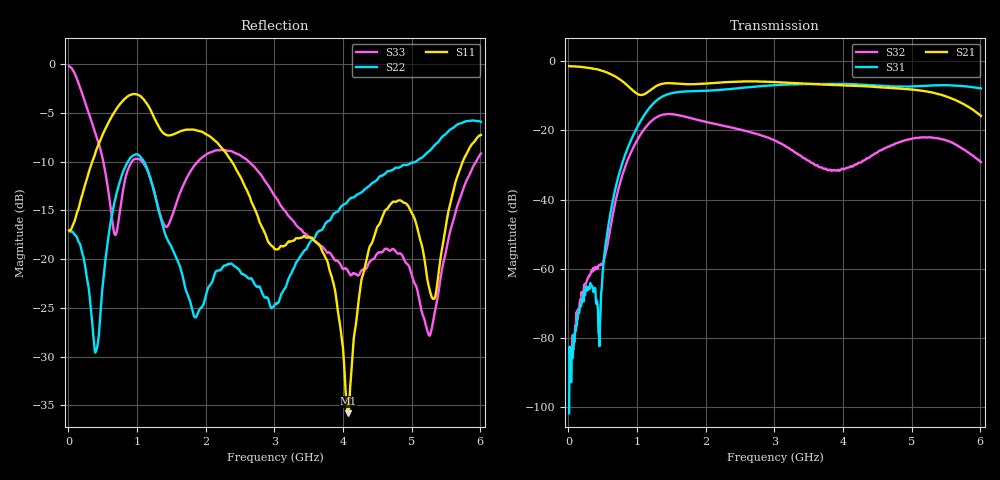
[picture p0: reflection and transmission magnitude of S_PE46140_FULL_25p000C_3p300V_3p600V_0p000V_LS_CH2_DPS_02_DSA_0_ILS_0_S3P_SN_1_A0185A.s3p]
! Device ID: PE46140_FULL
! File Path: z:\PE46140\MajorStates\25p000C\3p300\LS_CH2_DPS_02_DSA_0_ILS_0\PE46140_FULL_25p000C_3p300V_3p600V_0p000V_LS_CH2_DPS_02_DSA_0_ILS_0_S3P_SN_1_A0185A.s3p
! Serial: 1
! Lot: A0185A
! Temp: 25.000C
! VDD: 3.300
! VSS: 0.000
! Control_Hi: 3.600
! Control_Lo: 0.000
! Logic State: LS_CH2_DPS_02_DSA_0_ILS_0
! Port 1: RFIN
! Port 2: RFOUT1
! Port 3: RFOUT2
! ThroughPath:1-3
! IDD: 0.0003146759
! ISS: -1.196e-007
! Comment:
#  Hz  S  RI  R  50
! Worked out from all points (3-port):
!   801 points, 10 MHz to 6.01 GHz, reference 50 ohm
!   strongest paths, dB at 10 MHz, 1.51 GHz, 3.01 GHz, 4.51 GHz, 6.01 GHz:
!     S21: -1.5, -6.4, -6.1, -7.6, -15.9
!     S31: -101.7, -9.3, -7.0, -7.1, -7.9
!     S32: -84.2, -15.4, -23.0, -26.2, -29.2
!   lowest |S11| = -35.8 dB at 4.075 GHz (marker M1), VSWR 1.03, Z = 48.7 + j0.856 ohm
!   |S11| at or under -10 dB: start of sweep to 346.2 MHz; 2.382 GHz to 5.745 GHz (3.362 GHz wide, 82.7 % of centre)
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1e7  0.1401 -0.0109  0.842 -0.0246  -1.81e-05 -3.63e-05
     0.842 -0.0244  0.1399 -0.0067  4.69e-05 3.89e-05
     5.84e-06 -5.73e-06  5.97e-05 -1.44e-05  0.9746 -0.0929
3.4e8  -0.00118 -0.3117  0.4879 -0.6141  -0.000381 -0.00034
       0.4876 -0.6132  -0.000669 -0.0501  -0.000144 0.000854
       -0.000434 -0.000368  -0.000135 0.000897  -0.4192 -0.2818
4.525e8  -0.1196 -0.3793  0.2732 -0.6943  4.06e-05 0.000119
         0.2705 -0.6901  -0.0402 0.0204  0.000632 0.000889
         4.54e-05 6.13e-05  0.000541 0.000996  -0.3814 0.0132
7.075e8  -0.4708 -0.3661  -0.1594 -0.5548  0.0107 -0.0143
         -0.1586 -0.5557  0.102 0.1971  -0.00464 -0.0108
         0.0108 -0.0143  -0.00464 -0.0108  -0.1347 0.0392
1.195e9  -0.5188 0.2696  -0.2052 -0.3202  -0.1929 0.1034
         -0.2056 -0.3206  0.1665 -0.1985  0.0804 0.1046
         -0.1934 0.1035  0.0805 0.1046  0.0668 0.2497
3.01e9  0.0169 0.1111  0.4138 0.2744  -0.4079 -0.1863
        0.4136 0.2751  -0.0584 -0.00095  0.0595 -0.0381
        -0.4081 -0.1866  0.0594 -0.0381  0.1761 -0.1151
4.075e9  -0.0136 0.00879  0.00903 -0.4434  0.0561 0.4616
         0.00949 -0.4438  0.1498 0.1312  0.0276 0.00839
         0.0563 0.4614  0.0275 0.00859  0.0605 -0.0619
4.6225e9  -0.1659 -0.0678  -0.3758 -0.1712  0.3909 0.1888
          -0.3756 -0.1717  0.2715 0.0524  -0.037 -0.0408
          0.3915 0.1888  -0.0371 -0.0414  0.0815 -0.0783
5.2675e9  -0.0648 -0.023  -0.1672 0.3142  0.3528 -0.2661
          -0.1681 0.3137  0.3602 -0.0204  -0.00343 0.0784
          0.3532 -0.265  -0.00367 0.0785  0.0406 -0.00103
6.01e9  -0.3001 -0.3139  0.1532 0.0481  -0.2032 -0.3451
        0.1535 0.0485  0.2475 -0.4429  0.0293 -0.019
        -0.2045 -0.3462  0.0292 -0.0189  0.3167 0.1466
